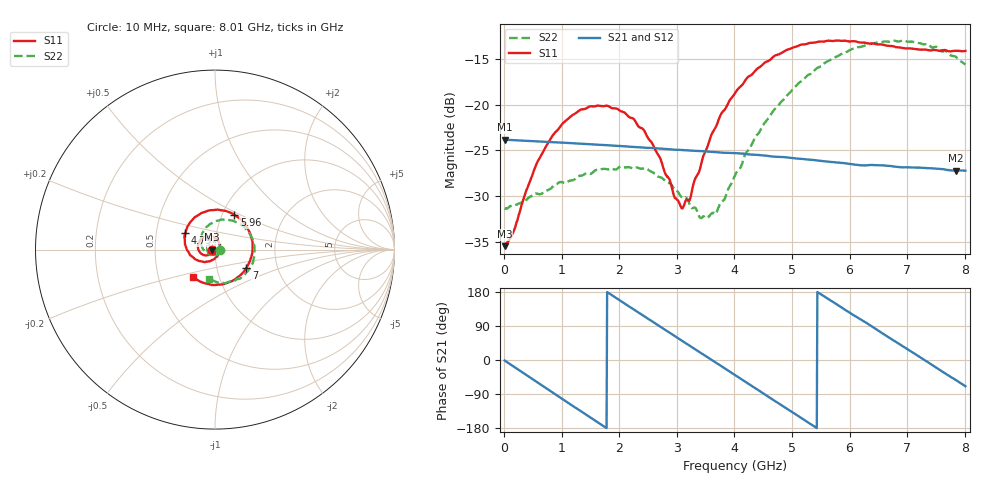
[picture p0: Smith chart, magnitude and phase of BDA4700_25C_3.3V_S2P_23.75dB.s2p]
!Agilent Technologies,E5071B,MY42404982,A.09.10
!Date: Mon Oct 20 18:13:02 2025
!Data & Calibration Information:
!Freq	S11:SOLT2(ON)	S21:SOLT2(ON)	S12:SOLT2(ON)	S22:SOLT2(ON)
# Hz S RI R 50
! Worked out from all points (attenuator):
!   801 points, 10 MHz to 8.01 GHz, reference 50 ohm
!   highest |S21| = -23.82 dB at 10 MHz (marker M1); lowest = -27.2 dB at 7.84 GHz (marker M2)
!   lowest |S11| = -35.4 dB at 10 MHz (marker M3), VSWR 1.03, Z = 48.3 - j0.0996 ohm
!   |S11| at or under -10 dB: start of sweep to end of sweep
!   |S22| runs from -32.4 to -13.0 dB; largest |S21 - S12| = 0.00074
!   S11 on the Smith chart (normalised r, x): 10 MHz: 0.97, -0.00; 4.79 GHz: 0.71, +0.14; 5.96 GHz: 1.14, +0.46; 7 GHz: 1.38, -0.30; 8.01 GHz: 0.75, -0.24
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1e7  -0.0169 -0.00103  0.0644 -0.00143  0.0644 -0.00147  0.0271 -0.000804
1.6e8  -0.0176 -0.00966  0.0612 -0.0183  0.0612 -0.0183  0.0272 -0.00769
5.3e8  -0.0342 -0.0288  0.0369 -0.0512  0.0369 -0.0512  0.0167 -0.0281
7.3e8  -0.0496 -0.0325  0.0168 -0.0603  0.0168 -0.0604  0.00414 -0.0337
1.35e9  -0.0942 0.00348  -0.0445 -0.0419  -0.0444 -0.0419  -0.0367 -0.0182
2.08e9  -0.054 0.0729  -0.0515 0.0292  -0.0515 0.0293  -0.03 0.0341
2.42e9  -0.011 0.0723  -0.0262 0.052  -0.0262 0.052  -0.0048 0.0446
2.68e9  0.0164 0.0503  -0.00102 0.0576  -0.00118 0.0575  0.0134 0.0382
2.96e9  0.0281 0.0135  0.0252 0.0508  0.0252 0.0507  0.0263 0.0229
3.1e9  0.0263 -0.0067  0.0366 0.0431  0.0363 0.0432  0.029 0.0113
3.23e9  0.0195 -0.0236  0.0448 0.0338  0.0448 0.0338  0.028 0.00228
3.54e9  -0.0149 -0.058  0.0551 0.00634  0.0551 0.00628  0.0139 -0.02
3.69e9  -0.0397 -0.066  0.0544 -0.00774  0.0545 -0.00787  0.00127 -0.0257
4.01e9  -0.0991 -0.0586  0.0418 -0.0346  0.0419 -0.0345  -0.0315 -0.0261
4.79e9  -0.1648 0.0929  -0.0233 -0.0463  -0.0229 -0.0464  -0.0784 0.0647
5.35e9  -0.0691 0.2059  -0.0494 -0.00716  -0.0493 -0.00746  -0.0158 0.1475
5.96e9  0.1086 0.193  -0.0298 0.0372  -0.0301 0.037  0.1224 0.1509
6.68e9  0.2088 -0.00456  0.0234 0.0399  0.0235 0.0399  0.22 -0.00103
7e9  0.1735 -0.1039  0.0397 0.0222  0.0397 0.022  0.2027 -0.0861
7.46e9  0.0504 -0.1919  0.0431 -0.0123  0.0432 -0.0122  0.1089 -0.1734
7.84e9  -0.0737 -0.1821  0.0266 -0.0345  0.0265 -0.0347  0.0107 -0.1822
8.01e9  -0.1217 -0.1538  0.0154 -0.0408  0.0156 -0.0407  -0.0313 -0.1622
